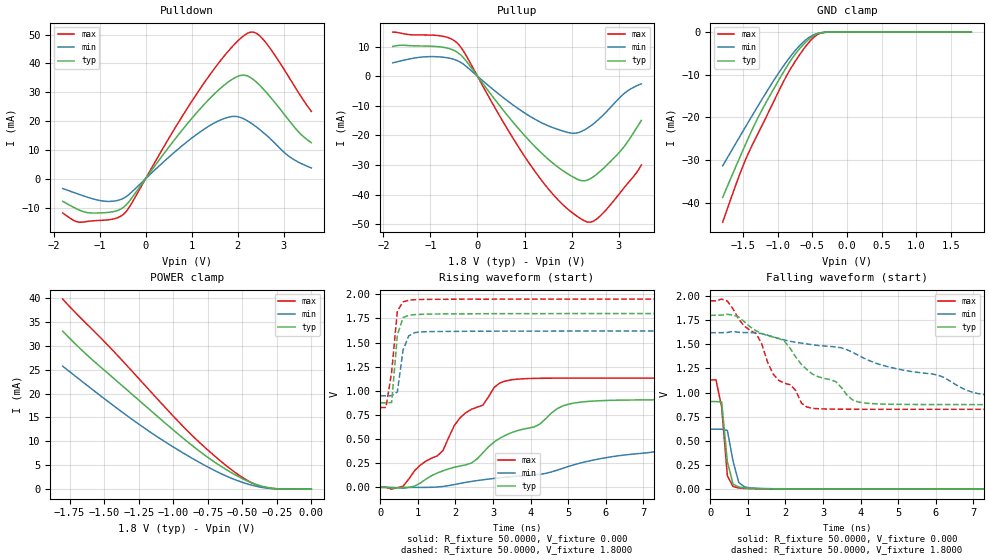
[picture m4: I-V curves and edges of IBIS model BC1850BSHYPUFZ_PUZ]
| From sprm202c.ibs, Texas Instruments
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|   Model BC1850BSHYPUFZ_PUZ
[Model]   BC1850BSHYPUFZ_PUZ
Model_type   I/O
Polarity   Non-Inverting
Enable   Active-Low
Vinl =   0.8500V
Vinh =   0.9800V
Vmeas =   0.9000V
Cref =  15.0000pF
Rref = 100.0000M
Vref =  0.000V
C_comp   1.2800pF   1.4600pF   1.1000pF
[Model Spec]
|   typ   min   max
Vinh   0.98V   0.86V   1.1V
Vinl   0.85V   0.70V   0.91V
[Temperature Range]   25.0000   0.1250k   -40.0000
[Voltage Range]   1.8000V   1.6200V   1.9500V
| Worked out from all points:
|   slope of the pulldown table from 0 to 0.27 V, typ, clamps not added: 45.4 ohm
|   slope of the pullup table from 0 to 0.27 V, typ, clamps not added: 46.7 ohm
|   GND clamp passes 1 mA (typ) near -0.50 V on its own axis
|   POWER clamp passes 1 mA (typ) near -0.40 V on its own axis
|   rising waveform, R_fixture 50.0000, V_fixture 0.000: 20-80 % time 2.69ns typ, 4.09ns min, 1.77ns max; typ from 0 V to 0.907 V
|   rising waveform, R_fixture 50.0000, V_fixture 1.8000: 20-80 % time 143ps typ, 185ps min, 186ps max; typ from 0.875 V to 1.8 V
|   falling waveform, R_fixture 50.0000, V_fixture 0.000: 20-80 % time 174ps typ, 212ps min, 163ps max; typ from 0.907 V to 0 V
|   falling waveform, R_fixture 50.0000, V_fixture 1.8000: 20-80 % time 2.11ns typ, 3.59ns min, 1.37ns max; typ from 1.8 V to 0.875 V
[Pulldown]
| voltage   I(typ)   I(min)   I(max)
-1.8V     -7.807mA   -3.392mA   -11.84mA
-1.44V    -10.87mA   -5.437mA   -15.06mA
-900mV    -11.77mA   -7.765mA   -14.36mA
-480mV    -9.903mA   -6.777mA   -12.32mA
720mV     15.38mA    10.45mA    19.67mA
1.38V     27.57mA    18.29mA    35.66mA
1.86V     34.25mA    21.54mA    45.38mA
2.22V     35.59mA    20mA       50.48mA
2.4V      33.61mA    18.03mA    50.48mA
2.58V     30.7mA     15.71mA    47.82mA
3.12V     20.13mA    7.698mA    35.04mA
3.6V      12.48mA    3.751mA    23.33mA
[Pullup]
| voltage   I(typ)   I(min)   I(max)
-1.8V     10.05mA    4.513mA    14.9mA
-1.08V    10.17mA    6.578mA    13.91mA
-660mV    9.559mA    6.262mA    13.21mA
-420mV    7.99mA     5.205mA    11.06mA
660mV     -13.69mA   -8.592mA   -18.48mA
1.2V      -23.44mA   -14.35mA   -31.7mA
1.92V     -33.02mA   -19.01mA   -44.92mA
2.28V     -35.33mA   -18.09mA   -48.94mA
2.46V     -33.99mA   -16.13mA   -49mA
2.64V     -31.65mA   -13.6mA    -46.71mA
3.12V     -23.67mA   -5.802mA   -37.58mA
3.48V     -14.97mA   -2.586mA   -30mA
[GND_clamp]
| voltage   I(typ)   I(min)   I(max)
-1.8V     -38.7mA    -31.3mA    -44.53mA
-1.6V     -31.11mA   -25.77mA   -35.33mA
-1.48V    -26.65mA   -22.47mA   -30.29mA
-1.32V    -21.05mA   -18.12mA   -24.75mA
-1.12V    -14.97mA   -12.84mA   -18.2mA
-920mV    -9.374mA   -7.926mA   -11.59mA
-760mV    -5.367mA   -4.511mA   -7.103mA
-600mV    -2.369mA   -1.843mA   -3.361mA
-480mV    -770.9uA   -620.5uA   -1.183mA
-400mV    -211.6uA   -201.1uA   -350.2uA
-280mV    -12.56uA   -20.13uA   -17.68uA
1.8V      13.13nA    8.713uA    2.416nA
[POWER_clamp]
| voltage   I(typ)   I(min)   I(max)
-1.8V     33.03mA    25.71mA    39.75mA
-1.6V     27.43mA    21.18mA    33.8mA
-1.42V    22.91mA    17.2mA     28.49mA
-1.12V    15.36mA    11.05mA    19.03mA
-960mV    11.42mA    8.12mA     14.07mA
-840mV    8.609mA    6.081mA    10.59mA
-720mV    6.046mA    4.196mA    7.435mA
-580mV    3.474mA    2.3mA      4.101mA
-440mV    1.421mA    904.2uA    1.469mA
-340mV    487.1uA    282.8uA    411.5uA
-220mV    51.94uA    24.5uA     37.88uA
0V        13.13nA    71.97nA    15.05nA
[Ramp]
| variable   typ   min   max
dV/dt_r   0.5191/2.6401n   0.1335/2.5015n   0.6787/1.7673n
dV/dt_f   0.5532/2.1510n   0.2266/2.3695n   0.6739/1.4100n
R_load = 50.0000
[Rising Waveform]
R_fixture = 50.0000
V_fixture = 0.000
V_fixture_min = 0.000
V_fixture_max = 0.000
| time   V(typ)   V(min)   V(max)
0s        9.213uV    8.989uV    8.92uV
606.1ps   -1.139mV   -8.874mV   11.39mV
1.061ns   43.42mV    -282.1uV   229.4mV
1.667ns   171mV      9.225mV    381.2mV
1.97ns    207.9mV    29.02mV    640.5mV
2.424ns   251.3mV    61.39mV    808mV
3.333ns   539.9mV    105.1mV    1.102V
5.455ns   887.8mV    264.4mV    1.131V
9.091ns   906.7mV    582.4mV    1.132V
15ns      906.8mV    620.2mV    1.132V
[Rising Waveform]
R_fixture = 50.0000
V_fixture = 1.8000
V_fixture_min = 1.6200
V_fixture_max = 1.9500
| time   V(typ)   V(min)   V(max)
0s        875.4mV    948.2mV    826.7mV
151.5ps   875.6mV    948.2mV    826.8mV
303ps     879.5mV    948.7mV    1.196V
454.5ps   1.579V     988.8mV    1.827V
606.1ps   1.758V     1.421V     1.921V
757.6ps   1.781V     1.569V     1.938V
909.1ps   1.789V     1.602V     1.943V
1.061ns   1.791V     1.609V     1.945V
1.515ns   1.795V     1.614V     1.947V
15ns      1.8V       1.62V      1.95V
[Falling Waveform]
R_fixture = 50.0000
V_fixture = 0.000
V_fixture_min = 0.000
V_fixture_max = 0.000
| time   V(typ)   V(min)   V(max)
0s        906.8mV    620.5mV    1.132V
151.5ps   906.8mV    620.5mV    1.131V
303ps     903.7mV    620.5mV    849.3mV
454.5ps   282.9mV    607.9mV    138.7mV
606.1ps   51.08mV    288.7mV    27.64mV
757.6ps   22.65mV    69.34mV    11.63mV
909.1ps   11.49mV    23.52mV    7.264mV
1.212ns   6.059mV    9.34mV     4.276mV
1.667ns   3.745mV    4.917mV    2.03mV
15ns      12.8uV     141.1uV    9.177uV
[Falling Waveform]
R_fixture = 50.0000
V_fixture = 1.8000
V_fixture_min = 1.6200
V_fixture_max = 1.9500
| time   V(typ)   V(min)   V(max)
0s        1.8V       1.62V      1.95V
454.5ps   1.81V      1.622V     1.947V
1.212ns   1.64V      1.619V     1.613V
1.667ns   1.574V     1.577V     1.195V
1.97ns    1.533V     1.545V     1.097V
2.727ns   1.189V     1.494V     836.7mV
3.333ns   1.115V     1.473V     828.2mV
3.939ns   902mV      1.385V     827.1mV
7.424ns   875.5mV    971.5mV    826.7mV
15ns      875.4mV    949.6mV    826.7mV
